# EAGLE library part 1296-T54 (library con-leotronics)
1.27mm SINGLE ROW FEMALE SOCKET Source: http://www.leotronics.co.uk/Conexcon/Data%20Sheets/sec.%20A/1296ing.pdf
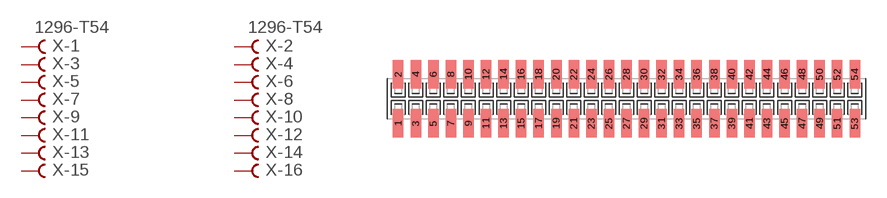
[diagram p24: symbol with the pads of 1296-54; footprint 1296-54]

Designator prefix X; gates -1=FVAL -2=FVAL -3=F -4=F -5=F -6=F -7=F -8=F -9=F -10=F -11=F -12=F -13=F -14=F -15=F -16=F -17=F -18=F -19=F -20=F -21=F -22=F -23=F -24=F -25=F -26=F -27=F -28=F -29=F -30=F -31=F -32=F -33=F -34=F -35=F -36=F -37=F -38=F -39=F -40=F -41=F -42=F -43=F -44=F -45=F -46=F -47=F -48=F -49=F -50=F -51=F -52=F -53=F -54=F

## 1296-T54 (OC_FARNELL: unknown; OC_NEWARK: unknown)  [1296-54]
1  -1:B  pas
2  -2:B  pas
3  -3:B  pas
4  -4:B  pas
5  -5:B  pas
6  -6:B  pas
7  -7:B  pas
8  -8:B  pas
9  -9:B  pas
10  -10:B  pas
11  -11:B  pas
12  -12:B  pas
13  -13:B  pas
14  -14:B  pas
15  -15:B  pas
16  -16:B  pas
17  -17:B  pas
18  -18:B  pas
19  -19:B  pas
20  -20:B  pas
21  -21:B  pas
22  -22:B  pas
23  -23:B  pas
24  -24:B  pas
25  -25:B  pas
26  -26:B  pas
27  -27:B  pas
28  -28:B  pas
29  -29:B  pas
30  -30:B  pas
31  -31:B  pas
32  -32:B  pas
33  -33:B  pas
34  -34:B  pas
35  -35:B  pas
36  -36:B  pas
37  -37:B  pas
38  -38:B  pas
39  -39:B  pas
40  -40:B  pas
41  -41:B  pas
42  -42:B  pas
43  -43:B  pas
44  -44:B  pas
45  -45:B  pas
46  -46:B  pas
47  -47:B  pas
48  -48:B  pas
49  -49:B  pas
50  -50:B  pas
51  -51:B  pas
52  -52:B  pas
53  -53:B  pas
54  -54:B  pas

## Footprint 1296-54 (pad centres in mm)
1.27mm SINGLE ROW FEMALE SOCKET Source: http://www.leotronics.co.uk/Conexcon/Data%20Sheets/sec.%20A/1296ing.pdf
smd 0.76 x 2.05: 1 -16.51,-1.78; 2 -16.51,1.78; 3 -15.24,-1.78; 4 -15.24,1.78; 5 -13.97,-1.78; 6 -13.97,1.78; 7 -12.7,-1.78; 8 -12.7,1.78; 9 -11.43,-1.78; 10 -11.43,1.78; 11 -10.16,-1.78; 12 -10.16,1.78; 13 -8.89,-1.78; 14 -8.89,1.78; 15 -7.62,-1.78; 16 -7.62,1.78; 17 -6.35,-1.78; 18 -6.35,1.78; 19 -5.08,-1.78; 20 -5.08,1.78; 21 -3.81,-1.78; 22 -3.81,1.78; 23 -2.54,-1.78; 24 -2.54,1.78; 25 -1.27,-1.78; 26 -1.27,1.78; 27 0,-1.78; 28 0,1.78; 29 1.27,-1.78; 30 1.27,1.78; 31 2.54,-1.78; 32 2.54,1.78; 33 3.81,-1.78; 34 3.81,1.78; 35 5.08,-1.78; 36 5.08,1.78; 37 6.35,-1.78; 38 6.35,1.78; 39 7.62,-1.78; 40 7.62,1.78; 41 8.89,-1.78; 42 8.89,1.78; 43 10.16,-1.78; 44 10.16,1.78; 45 11.43,-1.78; 46 11.43,1.78; 47 12.7,-1.78; 48 12.7,1.78; 49 13.97,-1.78; 50 13.97,1.78; 51 15.24,-1.78; 52 15.24,1.78; 53 16.51,-1.78; 54 16.51,1.78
